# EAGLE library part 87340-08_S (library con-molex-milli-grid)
RECEPTACAL
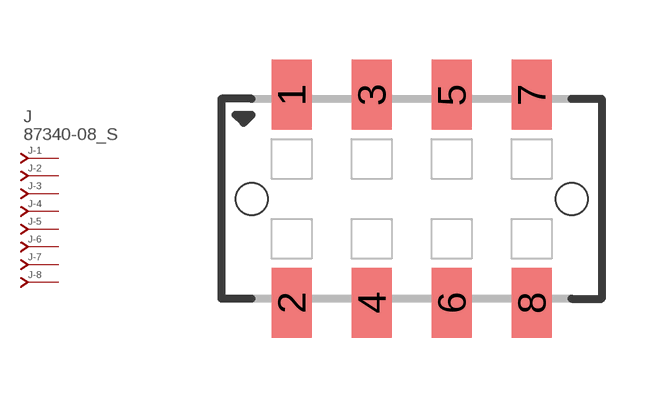
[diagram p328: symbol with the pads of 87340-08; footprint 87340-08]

Designator prefix J; gates -1=J-NV -2=J-N -3=J-N -4=J-N -5=J-N -6=J-N -7=J-N -8=J-N

## 87340-08_S  [87340-08]
1  -1:J  pas
2  -2:J  pas
3  -3:J  pas
4  -4:J  pas
5  -5:J  pas
6  -6:J  pas
7  -7:J  pas
8  -8:J  pas

## Footprint 87340-08 (pad centres in mm)
RECEPTACAL SMD Dual Row, Vertical, Low Profile
smd 1 x 1.75: 1 -3,2.6; 2 -3,-2.6; 3 -1,2.6; 4 -1,-2.6; 5 1,2.6; 6 1,-2.6; 7 3,2.6; 8 3,-2.6
hole 0.8 at -4,0
hole 0.8 at 4,0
